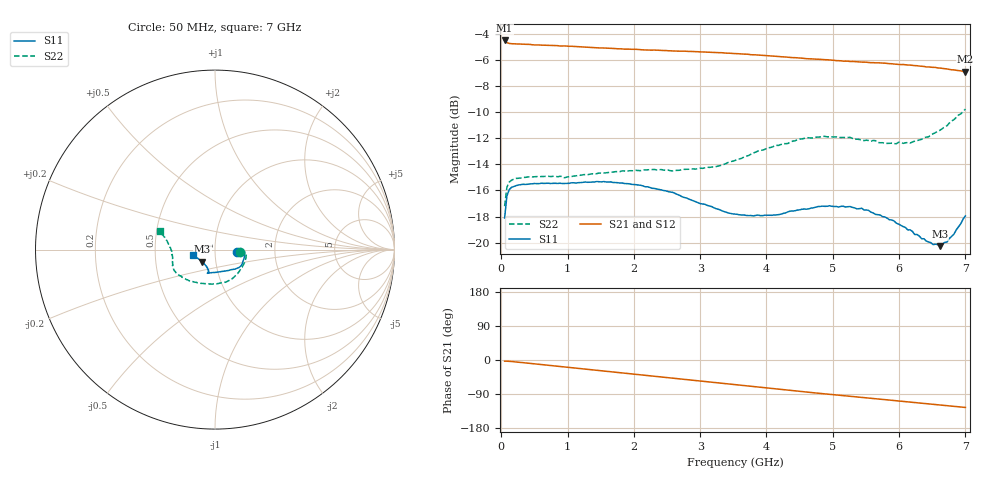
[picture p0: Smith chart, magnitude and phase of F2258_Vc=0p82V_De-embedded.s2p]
! Integrated Device Technology
! Corporate Headquarters
! 6024 Silver Creek Valley Road
! San Jose, CA 95138  USA
! Phone:  1-408-284-8200
! Toll Free:  1-800-223-1366
! Webpage:  http://www.idt.com/
! Timing and RF Division
! 515 Groton Road, Suite 102
! Westford, MA 01886-6024
! Device:  F2258
! Description: Voltage Variable RF Attenuator
! Frequency:  50.0 -  6000.00 MHz
! Package:  3x3 mm Thin QFN Plastic Package: 16 pin
! Ports:  2 RF, 2 DC
!  Pin  1  = NC
!  Pin  2  = NC
!  Pin  3  = RF2  = Port 2
!  Pin  4  = GND
!  Pin  5  = Vdd
!  Pin  6  = NC
!  Pin  7  = VCTRL
!  Pin  8  = NC
!  Pin  9  = GND
!  Pin 10  = RF1  = Port 1
!  Pin 11  = NC
!  Pin 12  = NC
!  Pin 13  = NC
!  Pin 14  = NC
!  Pin 15  = NC
!  Pin 16  = NC
! Vcntrl:  0.820 Volts
! Vdd:  +3.300 Volts
! Current:  1.135 mA
! Data:  The device was measured on a the F2258 evaluation board which has
!  individual transmission lines to the RF pins.  Data was collected
!  using a calibrated network analyzer.  The evaluation board was
!  de-embedded using a TRL calibration technique.
!  The reference plane is the edge of the package pin.
! Misc:  SN 10
!  Action Tracker AT0285
! Date Measured:  2014-12-10
! Date:  2016-01-13  MJV
! Note:
!  Integrated Device Technology supplies this data as a sample of measured
!  data at the package pin for this product.  Your particular data for this
!  product may vary.
!  Data was taken at 25 degrees C.
!  Integrated Device Technology reserves the right to change this data at anytime.
!Freq_(GHz)  S11M_(dB)  S11P_(deg)  S21M_(dB)  S21P_(deg)  S12M_(dB)  S12P_(deg)  S22M_(dB)  S22P_(deg)
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# GHz S dB R 50
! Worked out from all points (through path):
!   201 points, 50 MHz to 7 GHz, reference 50 ohm
!   highest |S21| = -4.47 dB at 50 MHz (marker M1); lowest = -6.9 dB at 7 GHz (marker M2)
!   group delay of S21, straight-line fit = 49.4 ps
!   lowest |S11| = -20.3 dB at 6.618 GHz (marker M3), VSWR 1.21, Z = 43.1 - j5.8 ohm
!   |S11| at or under -10 dB: start of sweep to end of sweep
!   |S22| runs from -17.2 to -9.7 dB; largest |S21 - S12| = 0.0019
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0.05  -18.12 -5.8  -4.47 -3.1  -4.46 -3.1  -17.21 -5.9
0.08475  -16.42 -4.0  -4.64 -3.1  -4.61 -3.1  -15.74 -4.8
0.1195  -15.94 -3.6  -4.70 -3.5  -4.67 -3.5  -15.36 -5.4
0.15425  -15.76 -4.1  -4.72 -4.0  -4.70 -4.0  -15.21 -6.6
0.6755  -15.45 -14.9  -4.84 -13.4  -4.84 -13.4  -14.91 -23.9
0.9535  -15.46 -21.6  -4.89 -18.6  -4.90 -18.6  -15.03 -34.1
1.2315  -15.38 -26.2  -4.97 -23.7  -4.98 -23.7  -14.79 -43.0
1.6485  -15.34 -32.1  -5.07 -31.2  -5.08 -31.2  -14.59 -54.9
2.37825  -15.92 -40.8  -5.22 -44.1  -5.24 -44.1  -14.40 -74.7
3.0385  -17.04 -54.4  -5.35 -56.2  -5.37 -56.1  -14.30 -96.9
3.525  -17.81 -71.4  -5.48 -65.2  -5.48 -65.2  -13.69 -116.3
4.081  -17.91 -92.9  -5.66 -75.4  -5.67 -75.4  -12.67 -135.5
4.498  -17.49 -103.9  -5.82 -82.8  -5.82 -82.8  -12.05 -146.3
4.7065  -17.33 -105.8  -5.89 -86.4  -5.91 -86.4  -11.96 -150.4
4.94975  -17.17 -107.2  -5.97 -90.6  -5.98 -90.6  -11.87 -154.4
5.43625  -17.37 -106.7  -6.13 -98.7  -6.15 -98.7  -12.13 -162.4
5.85325  -18.25 -107.3  -6.25 -105.7  -6.26 -105.8  -12.37 -170.8
6.166  -19.02 -111.7  -6.36 -111.1  -6.37 -111.1  -12.36 -178.0
6.33975  -19.71 -117.7  -6.45 -114.1  -6.46 -114.1  -12.07 177.2
6.61775  -20.28 -136.5  -6.59 -118.9  -6.59 -118.9  -11.37 169.9
6.82625  -19.37 -153.0  -6.73 -122.4  -6.74 -122.4  -10.56 165.1
7  -17.96 -166.2  -6.87 -125.2  -6.87 -125.3  -9.74 161.4
